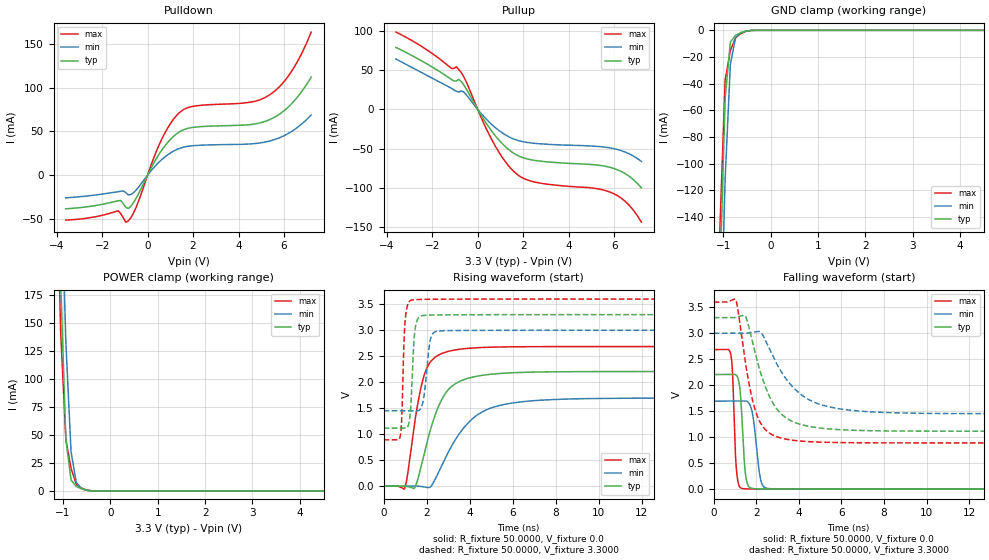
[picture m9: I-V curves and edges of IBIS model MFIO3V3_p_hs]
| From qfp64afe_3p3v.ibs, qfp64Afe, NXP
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[Model] MFIO3V3_p_hs
|   Model MFIO3V3_p_hs
| This model was characterised for following simulation conditions:
| External (pad) voltage:
|   - Typ: 3.3V,   - Min: 3.0V,   - Max: 3.6V
| Library cells for typ/min/max conditions are connected as defined below:
|  IO - External Pad
|  A - Core Input
|  EN - Output Buffer Enable
|  BOOST - vdde
|  EHS - vdd
|  ENZI - vdd
|  EPD - gnd
|  EPUN - vdd
|  ZI - NC
|  ZIF - NC
|  gnd - gnd
|  gnde - gnde
|  vdd - vdd
|  vdde - vdde
| All other pins connected to ground
Model_type I/O
Polarity   Non-Inverting
Enable   Active-Low
Vinl =   0.9900V
Vinh =   2.3100V
Vmeas =  1.6500V
Cref =   0.0F
Rref =   100.0000
Vref =   0.0V
C_comp   1.5616pF   1.4857pF   1.6280pF
|C_comp_pullup   0.7424pF   0.7664pF   0.7060pF
|C_comp_pulldown   0.6045pF   0.6430pF   0.5687pF
[Model Spec]
| variable   typ   min   max
Vinh   0.9900V   0.9000V   1.0800V
Vinl   2.3100V   2.1000V   2.5200V
Vmeas   1.6500V   1.5000V   1.8000V
[Temperature Range]   25.0000   0.1250k   -40.0000
[Voltage Range]   3.3000V   3.0000V   3.6000V
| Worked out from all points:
|   slope of the pulldown table from 0 to 0.495 V, typ, clamps not added: 21 ohm
|   slope of the pullup table from 0 to 0.495 V, typ, clamps not added: 21.7 ohm
|   GND clamp passes 1 mA (typ) near -0.56 V on its own axis
|   POWER clamp passes 1 mA (typ) near -0.54 V on its own axis
|   rising waveform, R_fixture 50.0000, V_fixture 0.0: 20-80 % time 1.06ns typ, 1.67ns min, 677ps max; typ from 0 V to 2.21 V
|   rising waveform, R_fixture 50.0000, V_fixture 3.3000: 20-80 % time 158ps typ, 234ps min, 125ps max; typ from 1.11 V to 3.3 V
|   falling waveform, R_fixture 50.0000, V_fixture 0.0: 20-80 % time 188ps typ, 278ps min, 145ps max; typ from 2.21 V to 0 V
|   falling waveform, R_fixture 50.0000, V_fixture 3.3000: 20-80 % time 1.14ns typ, 1.68ns min, 749ps max; typ from 3.3 V to 1.11 V
[Pulldown]
|Voltage   I(typ)   I(min)   I(max)
-3.6V     -38.54mA   -26.03mA   -51.47mA
-1.29V    -29.27mA   -18.96mA   -40.78mA
-960mV    -36.81mA   -20.01mA   -53.83mA
-850mV    -38.18mA   -22.68mA   -52.4mA
-520mV    -27.12mA   -17.5mA    -37.74mA
580mV     26.98mA    16.83mA    38.78mA
1.35V     48.62mA    30.01mA    70.27mA
2.01V     54.62mA    33.69mA    78.71mA
4.43V     57.57mA    35.54mA    83.11mA
5.31V     62.85mA    38.64mA    90.87mA
6.3V      80.67mA    49.35mA    117.4mA
7.2V      112.3mA    68.85mA    163.6mA
[Pullup]
|Voltage   I(typ)   I(min)   I(max)
-3.6V     79.43mA    64.59mA    99.03mA
-1.05V    36.46mA    25.05mA    52.51mA
-830mV    38.41mA    22.29mA    50.98mA
-610mV    31.13mA    22.16mA    41.54mA
270mV     -13.03mA   -9.075mA   -18mA
710mV     -31.29mA   -21.6mA    -43.53mA
1.26V     -48.73mA   -33.16mA   -68.54mA
1.7V      -58.01mA   -38.97mA   -82.27mA
2.58V     -65.44mA   -43.49mA   -93.28mA
5.88V     -74.5mA    -49.46mA   -106.4mA
6.65V     -85.19mA   -56.54mA   -122.1mA
7.2V      -100.2mA   -66.51mA   -144.2mA
[GND_clamp]
|Voltage   I(typ)   I(min)   I(max)
-3.6V     -4.776A    -4.755A    -4.803A
-1.07V    -185.2mA   -255.7mA   -147.9mA
-960mV    -51.25mA   -111.8mA   -37.35mA
-850mV    -8.87mA    -25.44mA   -15.18mA
-740mV    -3.773mA   -5.524mA   -5.635mA
-630mV    -1.795mA   -1.776mA   -2.434mA
-520mV    -584uA     -575.7uA   -771.5uA
-300mV    -2.698uA   -7.245uA   -2.257uA
7.2V      0A         0A         0A
[POWER_clamp]
|Voltage   I(typ)   I(min)   I(max)
-3.6V     5.691A     5.665A     5.731A
-1.16V    387.4mA    485.6mA    339.2mA
-1.05V    187.8mA    295.9mA    142.7mA
-940mV    46.35mA    133mA      46.17mA
-830mV    9.704mA    34.97mA    20.11mA
-720mV    3.968mA    7.718mA    5.953mA
-610mV    1.842mA    2.02mA     2.519mA
-500mV    572.5uA    622.5uA    738.7uA
-280mV    1.642uA    8.962uA    609.4nA
7.2V      0A         0A         0A
[Ramp]
| variable   typ   min   max
dV/dt_r  1.3236/1.0581n   1.0170/1.6720n   1.6117/0.6775n
dV/dt_f  1.3112/1.1412n   0.9294/1.6835n   1.6259/0.7490n
R_load = 50.0000
[Rising Waveform]
R_fixture= 50.0000
V_fixture= 0.0
V_fixture_min= 0.0
V_fixture_max= 0.0
|time   V(typ)   V(min)   V(max)
0s        3.927nV    110.6nV    42.16nV
985.7ps   60.11uV    -26.47uV   -34.52mV
1.464ns   -19.9mV    257.3uV    1.278V
1.787ns   452.1mV    -9.911mV   1.987V
2.131ns   1.022V     -26.22mV   2.364V
2.955ns   1.831V     610.1mV    2.587V
4.21ns    2.104V     1.323V     2.66V
6.002ns   2.182V     1.6V       2.682V
10.39ns   2.205V     1.689V     2.686V
100ns     2.206V     1.695V     2.686V
[Rising Waveform]
R_fixture= 50.0000
V_fixture= 3.3000
V_fixture_min= 3.0000
V_fixture_max= 3.6000
|time   V(typ)   V(min)   V(max)
0s        1.115V     1.451V     890.2mV
781.7ps   1.115V     1.451V     986.8mV
843.2ps   1.115V     1.451V     1.317V
976.3ps   1.113V     1.451V     3.045V
1.151ns   1.175V     1.451V     3.526V
1.456ns   2.998V     1.449V     3.589V
1.833ns   3.283V     1.63V      3.594V
2.215ns   3.293V     2.88V      3.596V
2.759ns   3.296V     2.99V      3.598V
100ns     3.3V       3V         3.6V
[Falling Waveform]
R_fixture= 50.0000
V_fixture= 0.0
V_fixture_min= 0.0
V_fixture_max= 0.0
|time   V(typ)   V(min)   V(max)
0s        2.206V     1.695V     2.686V
802.4ps   2.206V     1.695V     2.588V
882ps     2.207V     1.695V     2.226V
1.076ns   2.184V     1.695V     322.5mV
1.241ns   1.882V     1.695V     32.62mV
1.446ns   472.2mV    1.699V     7.816mV
1.8ns     14.29mV    1.493V     3.439mV
2.241ns   4.255mV    124mV      1.986mV
2.705ns   2.447mV    7.819mV    1.245mV
100ns     10.36nV    122nV      46.14nV
[Falling Waveform]
R_fixture= 50.0000
V_fixture= 3.3000
V_fixture_min= 3.0000
V_fixture_max= 3.6000
|time   V(typ)   V(min)   V(max)
0s        3.3V       3V         3.6V
1.046ns   3.308V     3V         3.631V
1.508ns   3.313V     3.002V     2.377V
1.852ns   2.781V     3.02V      1.659V
2.245ns   2.183V     3.004V     1.24V
3.04ns    1.503V     2.351V     998.3mV
4.314ns   1.222V     1.759V     918.2mV
6.343ns   1.137V     1.522V     894.6mV
10.32ns   1.116V     1.457V     890.2mV
100ns     1.115V     1.451V     890.2mV
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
